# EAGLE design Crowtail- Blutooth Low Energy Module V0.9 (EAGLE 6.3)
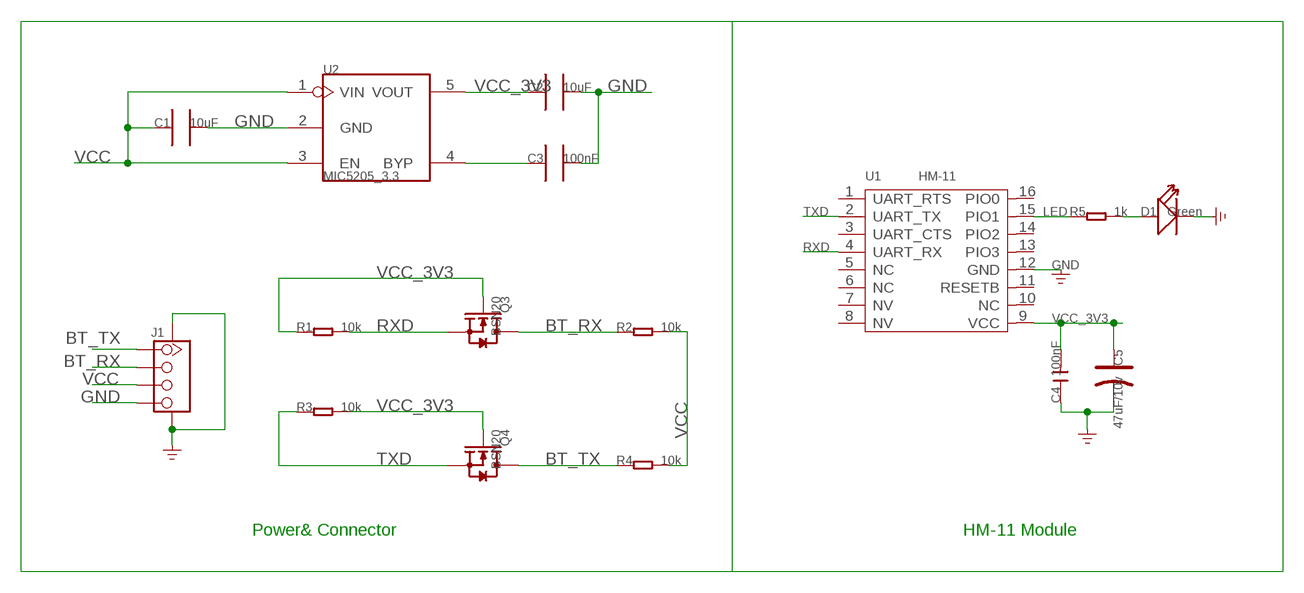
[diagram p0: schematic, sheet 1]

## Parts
C1  10uF  C0805_S  [0805_S]
C2  10uF  C0805_S  [0805_S]
C3  100nF  C0603_S  [0603_S]
C4  100nF  C-0603  [C0603]
C5  47uF/10v  CAP-AVX-B  [AVX-B]
D1  Green  LED'0603'  [LED-0603]
J1  TWIG-4P-2.0-SMD-FEMALE-REINFORCE'90D'  [4P-SMD-2.0-90D]
Q3  BSN20  MOSFET-N'SOT23'  [SOT23]
Q4  BSN20  MOSFET-N'SOT23'  [SOT23]
R1  10k  R-0603  [R0603]
R2  10k  R-0603  [R0603]
R3  10k  R-0603  [R0603]
R4  10k  R-0603  [R0603]
R5  1k  R-0603  [R0603]
U1  HM-11  [16P-18.5X13.5X0.8]
U2  MIC5205_3.3  MIC5025_X.X  [SOT23-5]

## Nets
BT_RX: J1.2 Q3.3(D) R2.1
BT_TX: J1.1 Q4.3(D) R4.1
GND: C1.2 C2.2 C3.2 C4.1 C5.- D1.- J1.4 J1.SS1 J1.SS2 U1.12(GND) U2.2(GND)
LED: R5.1 U1.15(PIO1)
N$3: C3.1 U2.4(BYP)
N$7: D1.+ R5.2
RXD: Q3.2(S) R1.2 U1.4(UART_RX)
TXD: Q4.2(S) R3.1 U1.2(UART_TX)
VCC: C1.1 J1.3 R2.2 R4.2 U2.1(VIN) U2.3(EN)
VCC_3V3: C2.1 C4.2 C5.+ Q3.1(G) Q4.1(G) R1.1 R3.2 U1.9(VCC) U2.5(VOUT)
Unconnected: U1.1(UART_RTS) U1.3(UART_CTS) U1.5(NC) U1.6(NC) U1.7(NV) U1.8(NV) U1.10(NC) U1.11(RESETB) U1.13(PIO3) U1.14(PIO2) U1.16(PIO0)

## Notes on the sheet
- Power& Connector | HM-11 Module

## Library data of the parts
C1 C2 = CPT_SMD:C0805
C3 = CPT_SMD:C0603
C4 = Discrete:C*: Ceramic Capacitors
C5 = Discrete:CAP*: Electrolytic Capacitors,Tantalum Capacitors and Super Capacitors
D1 = Discrete:LED*
J1 = Connector:TWIG-4P-2.0-SMD-FEMALE-REINFORCE
Q3 Q4 = Discrete:MOSFET-N: IRLL014: http://www.vishay.com/docs/91319/sihll014.pdf
R1-R5 = Discrete:R*
U1 = template:HM-11: Bluetooth Specification V4.0 BLE
U2 = ICs_v54:MIC5025_X.X

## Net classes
0 default: width 0.203 mm, drill 0.305 mm, clearance 0.203 mm

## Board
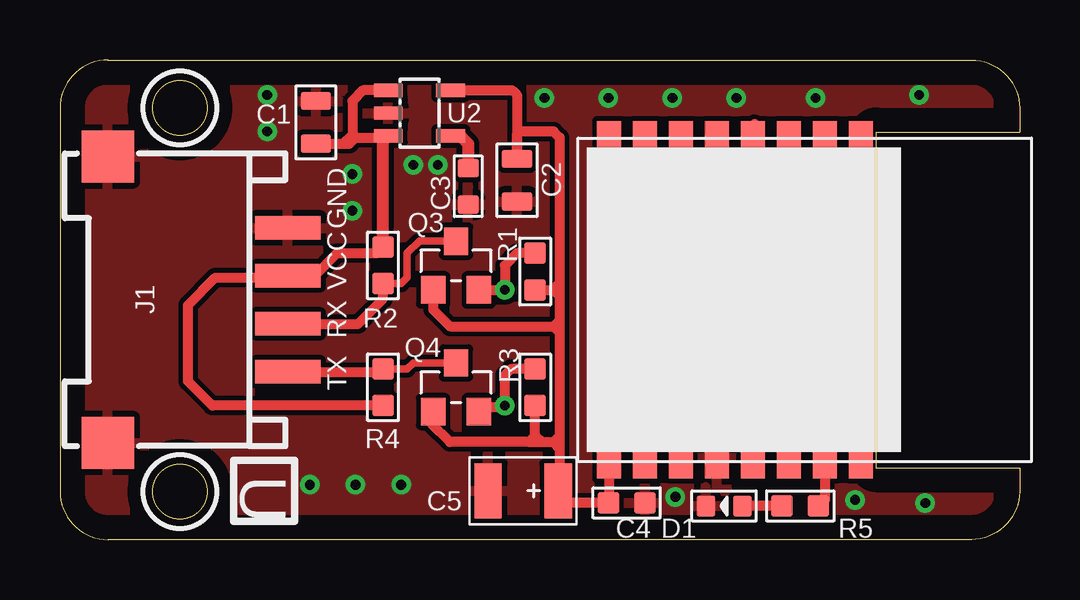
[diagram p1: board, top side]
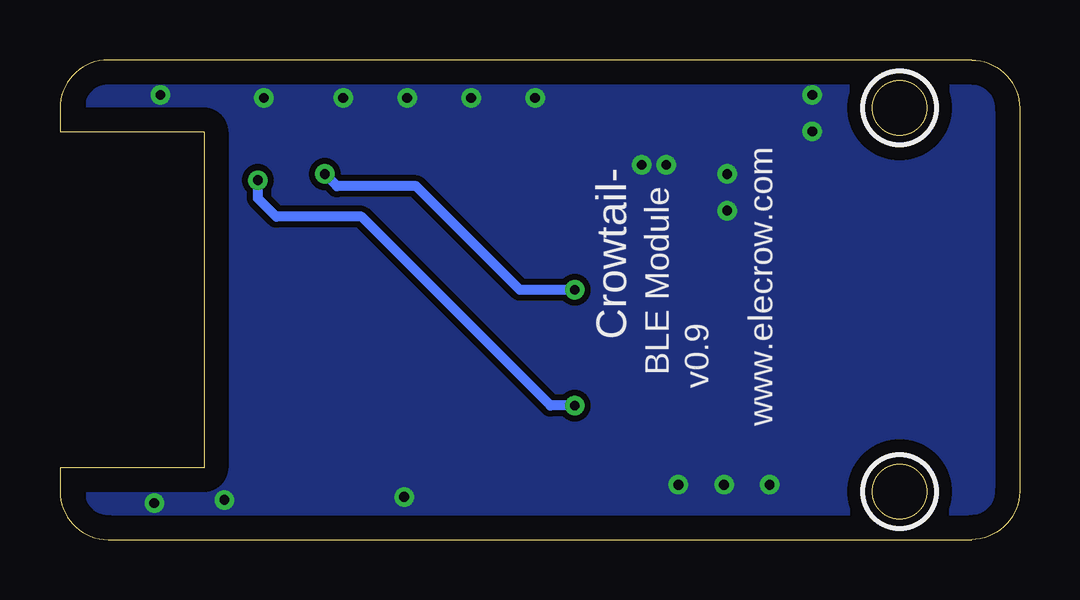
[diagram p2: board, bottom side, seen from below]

Size 40 x 20 mm. Coordinates in mm from the lower left corner, seen from the top.
Outline: 2,20 38,20 arc-90 40,18 40,17 34,17 34,3 40,3 40,2 arc-90 38,0 2,0 arc-90 0,2 0,18 arc-90 2,20
Outline: circle at 5,18 radius 1.14
Outline: circle at 5,2 radius 1.14
Copper layers (1*16): Top 0.035mm / dielectric 1.5mm / Bottom 0.035mm
Design rules "default *": minimum track width 10mil, minimum drill 24mil, track to track 8mil, track to pad 8mil, pad to pad 8mil, via to via 8mil, smd to smd 8mil, copper to edge 40mil, drill to drill 8mil, minimum pad ring 10mil, minimum via ring 8mil, stop-mask expansion 2mil, vias tented up to drill 100mil, thermal gap 10mil
tRestrict: area 3.5,16.5 to 6.5,19.5; area 3.5,0.5 to 6.5,3.5
bRestrict: area 3.5,16.5 to 6.5,19.5; area 3.5,0.5 to 6.5,3.5

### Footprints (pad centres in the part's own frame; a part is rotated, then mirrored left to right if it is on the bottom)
0805_S = smd 0.762 x 1.27: 1 -0.889,0; 2 0.889,0
0603_S = smd 0.762 x 0.889: 1 -0.762,0; 2 0.762,0
C0603 = smd 0.889 x 0.889: 1 -0.762,0; 2 0.762,0
AVX-B = smd 1.143 x 2.286: + -1.46,0; - 1.46,0
LED-0603 = smd 0.762 x 0.889: + -0.762,0; - 0.762,0
4P-SMD-2.0-90D = smd 0.965 x 2.74: 1 -3,-0.1; 2 -1,-0.1; 3 1,-0.1; 4 3,-0.1 | smd 2.159 x 2.184: SS1 -5.974,7.4; SS2 5.974,7.4
SOT23 = smd 1.016 x 1.143: 1 -0.95,-1.016; 2 0.95,-1.016; 3 0,1.016
R0603 = smd 0.889 x 0.889: 1 -0.762,0; 2 0.762,0
16P-18.5X13.5X0.8 = smd 1.7 x 1: 1 -6.6,2.15; 2 -6.6,0.65; 3 -6.6,-0.85; 4 -6.6,-2.35; 5 -6.6,-3.85; 6 -6.6,-5.35; 7 -6.6,-6.85; 8 -6.6,-8.35; 9 6.6,-8.35; 10 6.6,-6.85; 11 6.6,-5.35; 12 6.6,-3.85; 13 6.6,-2.35; 14 6.6,-0.85; 15 6.6,0.65; 16 6.6,2.15
SOT23-5 = smd 0.55 x 1.2: 1 -0.95,-1.3; 2 0,-1.3; 3 0.95,-1.3; 4 0.95,1.3; 5 -0.95,1.3

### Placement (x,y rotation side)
C1  10.67,17.4 90 top
C2  19.05,14.99 270 top
C3  17.02,14.73 270 top
C4  23.62,1.52 180 top
C5  19.3,2.03 180 top
D1  27.69,1.4 180 top
J1  9.4,10 90 top
Q3  16.51,11.43 0 top
Q4  16.51,6.35 0 top
R1  19.81,11.18 90 top
R2  13.46,11.43 90 top
R3  19.81,6.35 270 top
R4  13.46,6.35 270 top
R5  30.86,1.4 180 top
U1  31.24,10 270 top
U2  14.99,17.78 270 top

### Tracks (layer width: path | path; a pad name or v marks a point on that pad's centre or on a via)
BT_RX
  Top 0.305: R2.1 14.22,10.67 14.48,10.92 14.48,11.94 14.99,12.45 Q3.3
  Top 0.406: J1.2 12.43,9 13.46,10.03 R2.1
BT_TX
  Top 0.305: R4.1 14.48,7.11 14.73,7.37 Q4.3
  Top 0.406: J1.1 13.35,7 R4.1
GND  (via drill 0.41)
  other vias: 36.07,1.52 33.15,1.65 25.65,1.78 10.41,2.29 12.32,2.29 14.22,2.29 8.64,18.54 8.64,17.02 22.86,18.41 25.53,18.41 28.19,18.41 31.5,18.41 35.81,18.54 12.19,15.24 12.19,13.72 15.75,15.62 14.73,15.62 20.19,18.41
  pour Top: -1.27,20.32 41.91,20.32 41.91,0 -1.27,0
  pour Bottom (isolate 0.254): -1.27,20.32 41.91,20.32 41.91,0 -1.27,0
LED
  Top 0.406: U1.15 31.89,1.67 R5.1
N$3
  Top 0.508: U2.4 16.7,16.83 17.02,16.51 C3.1
N$7
  Top 0.406: R5.2 D1.+
RXD  (via drill 0.41)
  Top 0.406: U1.4 28.96,17.33 v28.96,15.24 | Q3.2 v18.54,10.41 18.54,11.43 19.05,11.94 R1.2
  Bottom 0.406: v28.96,15.24 28.45,14.73 25.15,14.73 20.83,10.41 v18.54,10.41
TXD  (via drill 0.41)
  Top 0.406: 17.53,5.33 Q4.2 17.46,5.52 18.22,5.52 18.29,5.59 v18.54,5.59 18.54,6.86 18.8,7.11 R3.1 | U1.2 31.75,17.25 v31.75,14.99
  Bottom 0.406: v31.75,14.99 31.75,14.22 30.99,13.46 27.43,13.46 19.56,5.59 v18.54,5.59
VCC
  Top 0.406: R4.2 6.35,5.59 5.33,6.6 5.33,9.78 6.48,10.92 9.42,10.92 J1.3 10.62,11 11.56,11.94 13.21,11.94 R2.2 | C1.1 11.81,16.51 | 11.81,16.51 12.06,16.51 12.32,16.76 13.62,16.76 | U2.1 12.63,18.73 12.19,18.29 12.19,16.89 11.81,16.51
  Top 0.508: R2.2 13.46,16.61 U2.3 13.62,16.76
VCC_3V3
  Top 0.406: 21.02,1.78 C5.+ | Q3.1 15.56,9.59 16.26,8.89 20.57,8.89 | 20.57,8.89 20.83,8.89 | 19.56,4.06 16.26,4.06 15.49,4.83 15.49,5.27 Q4.1 | U2.5 18.86,18.73 19.05,18.54 C2.1 19.05,16.89 19.18,17.02 20.57,17.02 20.83,16.76 20.83,10.67 | U1.9 22.89,1.56 C4.2 21.27,1.52 C5.+ | 20.83,10.67 20.83,10.16 | 20.83,10.16 20.83,9.14 | 20.83,9.14 20.83,8.89 | 20.83,8.89 20.83,8.64 | 20.83,8.64 20.83,4.32 | 20.83,4.32 20.83,4.06 | 20.83,4.06 20.83,3.81 | 20.83,3.81 20.83,2.1 C5.+ | 19.56,4.06 19.81,4.32 | 19.81,4.32 R3.2 | 19.56,4.06 20.07,4.06 | 20.57,4.06 20.83,4.06 | 19.81,4.32 20.07,4.06 | R1.1 20.57,10.41 | 20.57,10.41 20.83,10.16 | 20.83,10.67 20.57,10.41 | 20.83,9.14 20.57,8.89 | 20.57,8.89 20.83,8.64 | 20.57,4.06 20.83,4.32 | 20.07,4.06 20.57,4.06 | 20.57,4.06 20.83,3.81

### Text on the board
tPlace: GND | VCC | RX | TX | U
bPlace: www.elecrow.com | Crowtail- | BLE Module | v0.9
